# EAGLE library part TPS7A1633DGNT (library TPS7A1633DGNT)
Texas Instruments TPS7A1633DGNT, LDO Voltage Regulator, 100mA, 3.3 V +/-2%, 3 60 Vin, 8-Pin MSOP Source: Datasheet
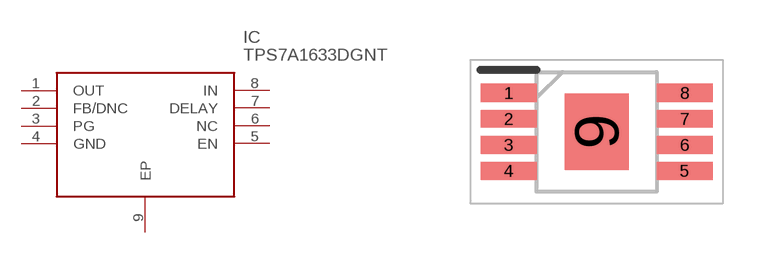
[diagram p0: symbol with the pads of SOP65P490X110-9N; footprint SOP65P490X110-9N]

Designator prefix IC

## TPS7A1633DGNT (Description: Texas Instruments TPS7A1633DGNT, LDO Voltage Regulator, 100mA, 3.3 V +/-2%, 3 60 Vin, 8-Pin MSOP; Height: 1.1mm; Manufacturer_Name: Texas Instruments; Manufacturer_Part_Number: TPS7A1633DGNT; Mouser_Part_Number: 595-TPS7A1633DGNT; Mouser_Price-Stock: https://www.mouser.co.uk/ProductDetail/Texas-Instruments/TPS7A1633DGNT?qs=KC2rBGieF4pkwFmfmKPfSg%3D%3D)  [SOP65P490X110-9N]
1  OUT
2  FB/DNC
3  PG
4  GND
5  EN
6  NC  nc
7  DELAY
8  IN
9  EP

## Footprint SOP65P490X110-9N (pad centres in mm)
DGN0008C
smd 1.4 x 0.45: 1 -2.2,0.975; 2 -2.2,0.325; 3 -2.2,-0.325; 4 -2.2,-0.975; 5 2.2,-0.975; 6 2.2,-0.325; 7 2.2,0.325; 8 2.2,0.975
smd 1.6 x 1.92: 9 0,0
